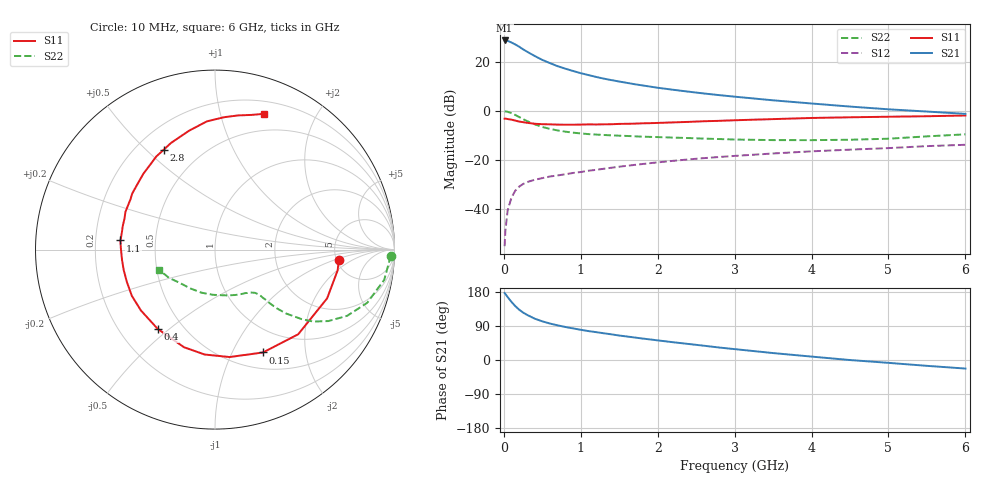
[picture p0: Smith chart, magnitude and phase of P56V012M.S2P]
! SIEMENS Small Signal Semiconductors
! BFP183
! Si NPN RF Bipolar Junction Transistor in SOT143
! VCE = 6 V  IC = 12 mA
! Common Emitter S-Parameters:  March  1996
# GHz  S  MA  R  50
!  f  S11  S21  S12  S22
! GHz  MAG  ANG  MAG  ANG  MAG  ANG  MAG  ANG
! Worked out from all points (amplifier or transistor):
!   36 points, 10 MHz to 6 GHz, reference 50 ohm
!   highest |S21| = 28.8 dB at 10 MHz (marker M1)
!   |S21| within 3 dB of that: start of sweep to 219.7 MHz
!   unconditionally stable (mu >= 1): 1.145 GHz to 5.675 GHz
!   at 250 MHz: K = 0.34, MSG = 27.6 dB, |S12| = -30.0 dB
!   at 1.4 GHz: K = 1.08, MAG = 16.2 dB, |S12| = -23.3 dB
!   at 6 GHz: K = 0.95, MSG = 6.3 dB, |S12| = -13.9 dB
!   S11 on the Smith chart (normalised r, x): 10 MHz: 5.25, -1.12; 150 MHz: 0.69, -1.32; 400 MHz: 0.36, -0.46; 1.1 GHz: 0.31, +0.04; 2.8 GHz: 0.31, +0.57; 6 GHz: 0.32, +1.37
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0.01  0.6922 -4.6  27.65 176.9  0.0017 84.7  0.9808 -2.0
0.02  0.693 -9.6  27.52 174.4  0.0035 85.4  0.9722 -4.1
0.05  0.6812 -23.5  27.12 165.9  0.0093 81.1  0.958 -10.1
0.1  0.6614 -45.5  25.07 153.1  0.0169 68.2  0.8982 -19.3
0.15  0.6324 -65.0  22.84 141.9  0.0234 61.3  0.8236 -26.6
0.2  0.6041 -82.3  20.53 132.7  0.0282 56.0  0.7471 -32.2
0.25  0.5874 -95.6  18.19 125.2  0.0318 52.5  0.679 -36.2
0.3  0.5707 -107.6  16.34 119.3  0.0348 49.1  0.6204 -38.7
0.4  0.5452 -125.8  13.32 109.2  0.0389 45.5  0.5313 -42.0
0.5  0.5342 -140.6  11.05 102.0  0.042 43.8  0.4687 -43.7
0.6  0.5302 -150.9  9.498 96.2  0.0454 43.7  0.4275 -44.4
0.7  0.5231 -159.9  8.213 91.4  0.0477 43.3  0.3975 -44.7
0.9  0.5212 -173.8  6.557 83.4  0.0536 44.0  0.3585 -45.4
1.1  0.5291 174.5  5.409 76.3  0.0596 44.8  0.3347 -46.7
1.5  0.5414 157.3  3.988 64.6  0.072 45.3  0.3106 -50.4
1.8  0.5569 146.0  3.325 56.7  0.0816 45.1  0.2965 -54.7
2.2  0.5812 133.4  2.707 46.9  0.0949 43.5  0.2839 -61.5
2.8  0.6255 117.2  2.101 32.9  0.1137 39.9  0.2651 -74.5
3.5  0.6784 102.2  1.645 18.3  0.1343 35.2  0.2522 -92.5
4.5  0.7393 86.1  1.225 -0.1  0.1608 27.4  0.2567 -123.0
5.5  0.7772 74.9  0.969 -15.4  0.1899 20.5  0.3009 -148.5
6  0.8038 70.2  0.869 -22.6  0.2022 16.2  0.331 -160.0
